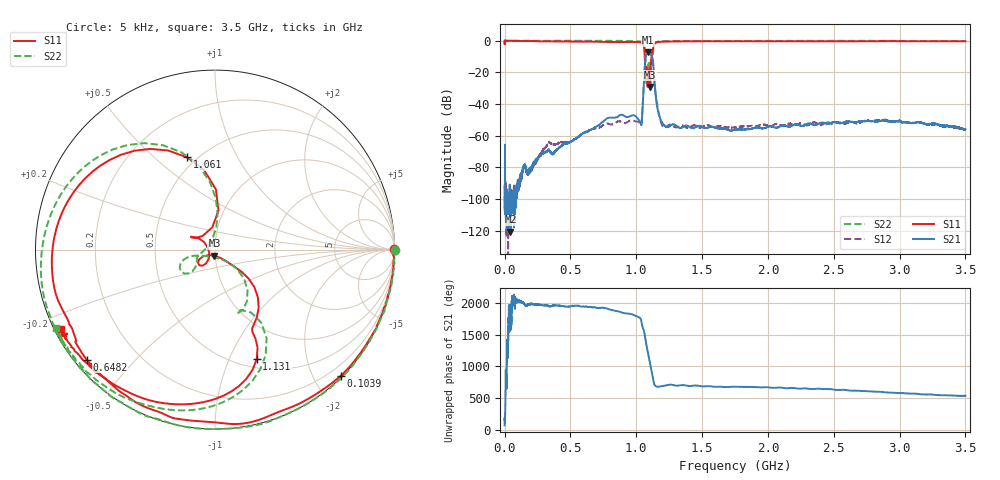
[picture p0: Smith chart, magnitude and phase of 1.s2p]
#  HZ  S  MA  R  50.00
! Rohde & Schwarz Vector Network Analyzer
! Rohde-Schwarz,ZNL6-2Port,1323001206101378,1.50.1.34-21.10.1.104
! Created: UTC 12/25/2023, 3:41:10 AM
! freq[Hz]  mag:S11  ang:S11  mag:S21  ang:S21  mag:S12  ang:S12  mag:S22  ang:S22
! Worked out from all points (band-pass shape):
!   6000 points, 5 kHz to 3.5 GHz, reference 50 ohm
!   highest |S21| = -7.27 dB at 1.089 GHz (marker M1); lowest = -120.7 dB at 44.35 MHz (marker M2)
!   |S21| within 3 dB of the highest: 1.071 GHz to 1.121 GHz (50.38 MHz wide, 4.6 % of centre)
!   lowest |S11| = -29.3 dB at 1.103 GHz (marker M3), VSWR 1.07, Z = 49.6 - j3.41 ohm
!   |S11| at or under -10 dB: 1.064 GHz to 1.115 GHz (50.91 MHz wide, 4.67 % of centre)
!   |S22| runs from -27.3 to 0.2 dB; largest |S21 - S12| = 0.027
!   S11 on the Smith chart (normalised r, x): 5 kHz: open; 103.9 MHz: 0.03, -2.40; 648.2 MHz: 0.03, -0.37; 1.061 GHz: 0.44, +0.64; 1.131 GHz: 0.60, -1.27; 3.5 GHz: 0.02, -0.24
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5000  0.9983 0.2  4.588e-06 71.8  2.641e-05 81.7  1.002 -0.1
4.434566e7  0.9978 -20.0  9.184e-07 48.4  1.766e-06 25.2  1.002 -20.2
1.038555e8  0.992 -45.2  2.361e-05 -139.4  3.013e-05 -138.3  1.004 -45.1
2.112066e8  0.9815 -80.8  0.0001185 179.8  0.0001081 -175.2  1.003 -80.1
3.331434e8  0.9655 -105.0  0.0003649 150.7  0.0006172 122.9  0.9959 -107.5
5.834347e8  0.9406 -137.4  0.001103 136.8  0.001108 124.6  1.001 -133.7
6.481954e8  0.9418 -139.4  0.001486 132.4  0.001483 110.6  0.9948 -139.2
8.827342e8  0.9088 -154.4  0.004581 51.8  0.002791 30.1  0.9955 -153.1
9.80167e8  0.9202 -166.6  0.0044 8.0  0.00301 -4.8  0.9874 -166.1
1.025674e9  0.8976 175.5  0.002877 -34.5  0.002571 -38.6  0.959 177.7
1.042011e9  0.8539 159.0  0.002617 -129.2  0.003153 -149.2  0.9233 163.7
1.06068e9  0.5376 106.8  0.08291 95.6  0.07683 89.7  0.7122 123.6
1.074683e9  0.1524 152.3  0.3686 -76.4  0.366 -78.7  0.06407 101.8
1.089268e9  0.07318 -122.3  0.433 125.9  0.4304 123.4  0.1806 -136.4
1.102687e9  0.03443 -95.0  0.4181 -8.9  0.421 -10.7  0.1226 -163.9
1.130692e9  0.6512 -69.1  0.1459 42.4  0.1358 44.8  0.5727 -59.8
1.166864e9  0.9127 -112.4  0.005618 -40.1  0.006254 -49.3  0.9416 -111.6
1.214122e9  0.9403 -127.5  0.002076 -24.5  0.001813 -20.9  0.9753 -127.5
1.750294e9  0.9705 -149.1  0.001551 -39.9  0.001821 -47.4  0.9887 -147.3
2.333724e9  0.9622 -150.5  0.002299 -76.5  0.002508 -80.2  0.9935 -149.0
2.917154e9  0.9769 -150.7  0.002837 -131.6  0.003035 -133.5  0.991 -150.6
3.5e9  0.9633 -152.6  0.001582 178.0  0.001535 -176.7  0.9854 -153.9
